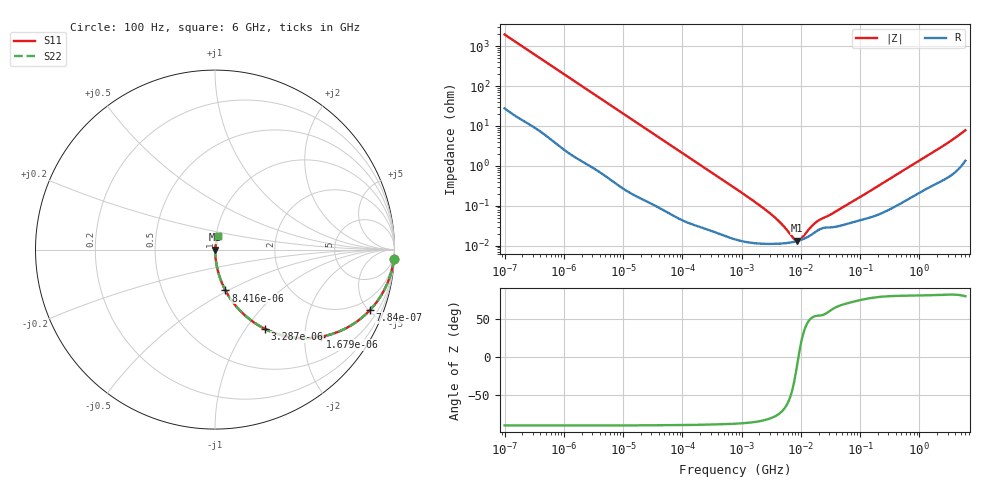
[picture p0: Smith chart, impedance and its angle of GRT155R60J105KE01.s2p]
!Murata Part Number: GRT155R60J105KE01
!These Parameters are Measured in Series Mode Connection
!Data Generated on Jun 19, 2026
!  o--ll--o
!Port1  Port2
!  o------o
!Operation Temp=25[degC], DC Bias Voltage=0[V]
!Freq. Start=100[Hz] Stop=6[GHz] 401[Steps]
# Hz S RI R 50
!Freq.(Hz) S11(Real) S11(Imag) S21(Real) S21(Imag) S12(Real) S12(Imag) S22(Real) S22(Imag)
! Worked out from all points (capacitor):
!   401 points, 100 Hz to 6 GHz, reference 50 ohm
!   read as one part in series: C = 808 nF near 109 Hz
!   lowest |Z| = 13.1 mohm at 8.692 MHz (marker M1)
!   series resonance near 9.106 MHz, so ESL is about 380 pH
!   S11 on the Smith chart (normalised r, x): 100 Hz: 2, -39; 784 Hz: 1.07, -5.10; 1.679 kHz: 1.03, -2.39; 3.287 kHz: 1.02, -1.23; 8.416 kHz: 1.01, -0.48; 6 GHz: 1.03, +0.15
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100  0.9967 -0.0507  0.0033 0.0507  0.0033 0.0507  0.9967 -0.0507
293  0.9766 -0.1441  0.0234 0.1441  0.0234 0.1441  0.9766 -0.1441
784  0.8635 -0.3368  0.1365 0.3368  0.1365 0.3368  0.8635 -0.3368
1122  0.7587 -0.4216  0.2413 0.4216  0.2413 0.4216  0.7587 -0.4216
1679  0.588 -0.4859  0.412 0.4859  0.412 0.4859  0.588 -0.4859
2008  0.5012 -0.4936  0.4988 0.4936  0.4988 0.4936  0.5012 -0.4936
3287  0.2773 -0.4409  0.7227 0.4409  0.7227 0.4409  0.2773 -0.4409
5143  0.1382 -0.3384  0.8618 0.3384  0.8618 0.3384  0.1382 -0.3384
8416  0.0581 -0.2274  0.9419 0.2274  0.9419 0.2274  0.0581 -0.2274
17227  0.0155 -0.1168  0.9845 0.1168  0.9845 0.1168  0.0155 -0.1168
40335  0.00349 -0.051  0.9965 0.051  0.9965 0.051  0.00349 -0.051
774597  0.00015 -0.00274  0.9998 0.00274  0.9998 0.00274  0.00015 -0.00274
3245845  0.00011 -0.000578  0.9999 0.000578  0.9999 0.000578  0.00011 -0.000578
4856642  0.000113 -0.000316  0.9999 0.000316  0.9999 0.000316  0.000113 -0.000316
7599586  0.000123 -8.52e-05  0.9999 8.52e-05  0.9999 8.52e-05  0.000123 -8.52e-05
8692127  0.00013 -2.17e-05  0.9999 2.17e-05  0.9999 2.17e-05  0.00013 -2.17e-05
1.039699e7  0.000141 6.16e-05  0.9999 -6.16e-05  0.9999 -6.16e-05  0.000141 6.16e-05
1.555665e7  0.000192 0.000248  0.9998 -0.000248  0.9998 -0.000248  0.000192 0.000248
2.035112e7  0.000251 0.000354  0.9997 -0.000354  0.9997 -0.000354  0.000251 0.000354
3.482834e7  0.000289 0.000579  0.9997 -0.000579  0.9997 -0.000579  0.000289 0.000579
3.124326e8  0.000818 0.00458  0.9992 -0.00458  0.9992 -0.00458  0.000818 0.00458
6e9  0.0189 0.0743  0.9811 -0.0743  0.9811 -0.0743  0.0189 0.0743
